(* Logix 5000 AddOnInstructionDefinition export YAI_Assy_170_22_23_EIP_Hz; software revision 21.03 *)

ADD_ON_INSTRUCTION YAI_Assy_170_22_23_EIP_Hz   (* revision 1.0, vendor Yaskawa America, Inc. *)
// YAI Assembly 170 and 22/23
// Help:
// This add-on instruction is for use with input assembly 170 and output assemblies 22/23.
// Node_Input_Assy is defined as the node's input assembly integer array.
// Node_Output_Assy is defined as the node's output assembly integer array.
// Torque limit/reference, torque compensation and torque output variables are only available with A1000.
VAR_IN_OUT
   Node_Input_Assy : AB:ETHERNET_MODULE_INT_24Bytes:I:0; {required}   // Input assembly words
   Node_Output_Assy : AB:ETHERNET_MODULE_INT_6Bytes:O:0; {required}   // Output assembly words
END_VAR
VAR_OUTPUT
   Running : BOOL; {access Read Only, visible}   // Drive running forward status bit
   ZSP : BOOL; {access Read Only, visible}   // Drive zero speed status bit
   RunningRev : BOOL; {access Read Only, visible}   // Drive running reverse status bit
   Reset : BOOL; {access Read Only, visible}   // Drive reset command status bit
   At_Speed : BOOL; {access Read Only, visible}   // Drive at commanded speed status bit
   Ready : BOOL; {access Read Only, visible}   // Drive ready status bit
   Alarm : BOOL; {access Read Only, visible}   // Drive alarm status bit
   Faulted : BOOL; {access Read Only, visible}   // Drive faulted status bit
   OPE : BOOL; {access Read Only}   // OPE alarm/fault present
   UV : BOOL; {access Read Only}   // Drive in UV (undervoltage) state status bit
   NetCtrlStatus : BOOL; {access Read Only, visible}   // Drive network run source status bit (1 = source coming from network)
   MFO_1_Status : BOOL; {access Read Only, visible}   // Drive multi-function output 1 (M1-M2 for A/P1000, MA/MB/MC for V1000) status
   MFO_2_Status : BOOL; {access Read Only, visible}   // Drive multi-function output 1 (M3-M4 for A/P1000, P1 for V1000) status
   MFO_3_Status : BOOL; {access Read Only, visible}   // Drive multi-function output 1 (M5-M6 for A/P1000, P2 for V1000) status
   ZSV : BOOL; {access Read Only, visible}   // Drive zero servo completed status bit
   Motor_Speed : REAL; {access Read Only, visible}   // Motor speed in Hz (xx.xx resolution)
   Custom_In_1 : INT; {access Read Only}
   Custom_In_2 : INT; {access Read Only}
   Custom_In_3 : INT; {access Read Only}
   Custom_In_4 : INT; {access Read Only}
   Custom_In_5 : INT; {access Read Only}
   Custom_In_6 : INT; {access Read Only}
   Custom_In_7 : INT; {access Read Only}
   Custom_In_8 : INT; {access Read Only}
   Custom_In_9 : INT; {access Read Only}
   Custom_In_10 : INT; {access Read Only}
END_VAR
VAR_INPUT
   Torq_Ref_Limit : REAL; {visible}   // Torque reference/limit (A1000 only) Engineering Units
   RunRev : BOOL; {visible}   // Reverse run command
   RunFwd : BOOL; {visible}   // Forward run command
   Net_Ref : BOOL;   // Network reference bit to switch between b1-01 setting and network.
   Net_Control : BOOL;   // Network control bit to switch between b1-02 setting and network.
   Motor_Rated_Torq : REAL := 100.0; {visible}   // Motor rated torque (Engineering units)
   Freq_Ref : REAL; {visible}   // Frequency reference command in Hz (xx.xx resolution)
   FaultReset : BOOL; {visible}   // Fault reset command
END_VAR
VAR
   FRef_Convert : DINT;
   FOut_Convert : REAL;
   FOut_Temp : REAL;
   TRef_Convert : INT;
   TComp_Convert : INT;
   TOut_Convert : REAL;
   TOut_Temp : REAL;
   IOut_Temp : REAL;
   IOut_Convert : REAL;
   AO1_Convert : INT;
   AO2_Convert : INT;
   Motor_Speed_Temp : REAL;
   Motor_Speed_Convert : REAL;
   Freq_Cmd_Temp : REAL;
   Freq_Cmd_Convert : REAL;
   AI1_Temp : REAL;
   AI1_Convert : REAL;
   AI2_Temp : REAL; {access None}
   AI2_Convert : REAL; {access None}
   AI3_Temp : REAL; {access None}
   AI3_Convert : REAL; {access None}
END_VAR

ROUTINE Logic   (* ladder *)
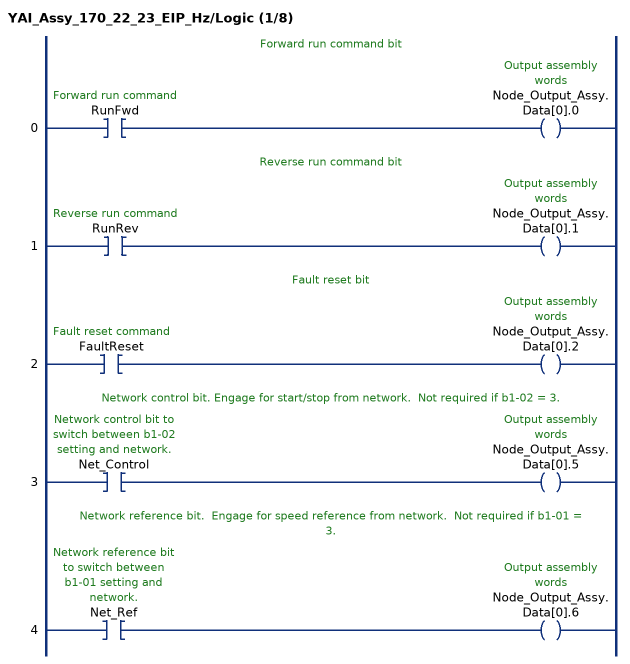
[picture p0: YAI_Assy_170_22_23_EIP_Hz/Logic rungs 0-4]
   // Forward run command bit
   0: XIC(RunFwd)OTE(Node_Output_Assy.Data[0].0);
   // Reverse run command bit
   1: XIC(RunRev)OTE(Node_Output_Assy.Data[0].1);
   // Fault reset bit
   2: XIC(FaultReset)OTE(Node_Output_Assy.Data[0].2);
   // Network control bit. Engage for start/stop from network.  Not required if b1-02 = 3.
   3: XIC(Net_Control)OTE(Node_Output_Assy.Data[0].5);
   // Network reference bit.  Engage for speed reference from network.  Not required if b1-01 = 3.
   4: XIC(Net_Ref)OTE(Node_Output_Assy.Data[0].6);
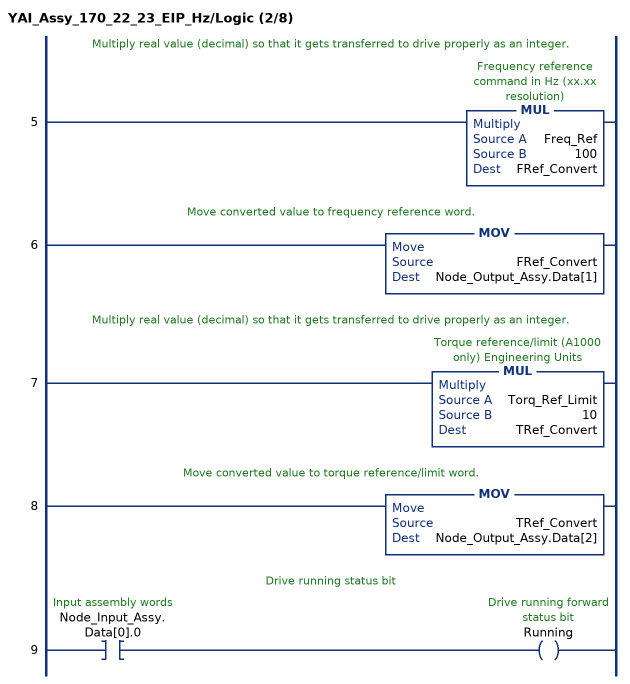
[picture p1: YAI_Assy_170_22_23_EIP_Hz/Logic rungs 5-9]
   // Multiply real value (decimal) so that it gets transferred to drive properly as an integer.
   5: MUL(Freq_Ref,100,FRef_Convert);
   // Move converted value to frequency reference word.
   6: MOV(FRef_Convert,Node_Output_Assy.Data[1]);
   // Multiply real value (decimal) so that it gets transferred to drive properly as an integer.
   7: MUL(Torq_Ref_Limit,10,TRef_Convert);
   // Move converted value to torque reference/limit word.
   8: MOV(TRef_Convert,Node_Output_Assy.Data[2]);
   // Drive running status bit
   9: XIC(Node_Input_Assy.Data[0].0)OTE(Running);
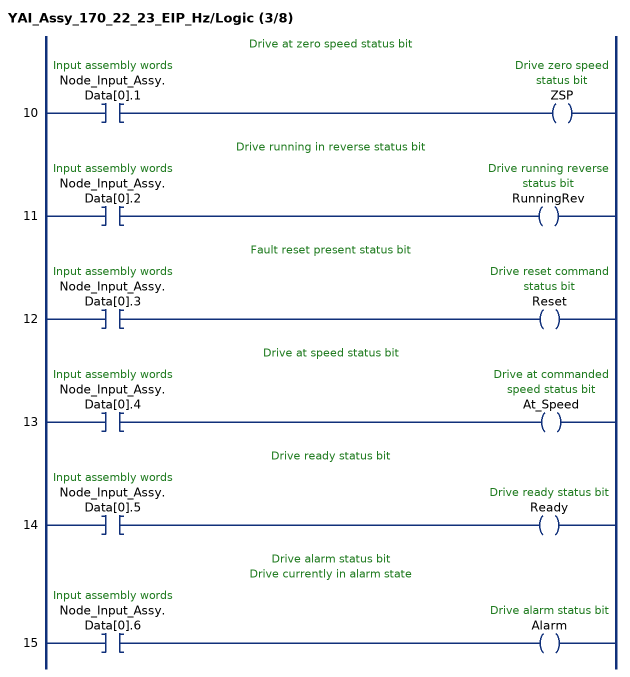
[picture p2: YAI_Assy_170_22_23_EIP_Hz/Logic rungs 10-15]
   // Drive at zero speed status bit
   10: XIC(Node_Input_Assy.Data[0].1)OTE(ZSP);
   // Drive running in reverse status bit
   11: XIC(Node_Input_Assy.Data[0].2)OTE(RunningRev);
   // Fault reset present status bit
   12: XIC(Node_Input_Assy.Data[0].3)OTE(Reset);
   // Drive at speed status bit
   13: XIC(Node_Input_Assy.Data[0].4)OTE(At_Speed);
   // Drive ready status bit
   14: XIC(Node_Input_Assy.Data[0].5)OTE(Ready);
   // Drive alarm status bit
   // Drive currently in alarm state
   15: XIC(Node_Input_Assy.Data[0].6)OTE(Alarm);
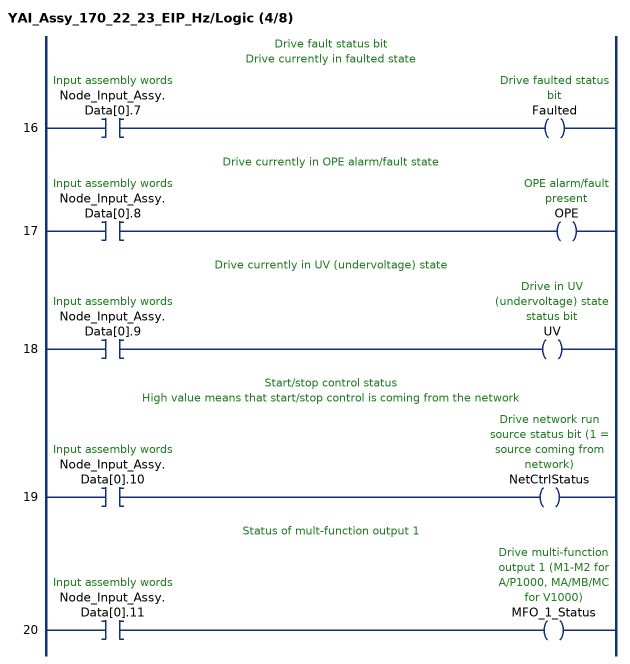
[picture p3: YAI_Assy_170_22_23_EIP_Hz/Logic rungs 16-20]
   // Drive fault status bit
   // Drive currently in faulted state
   16: XIC(Node_Input_Assy.Data[0].7)OTE(Faulted);
   // Drive currently in OPE alarm/fault state
   17: XIC(Node_Input_Assy.Data[0].8)OTE(OPE);
   // Drive currently in UV (undervoltage) state
   18: XIC(Node_Input_Assy.Data[0].9)OTE(UV);
   // Start/stop control status
   // High value means that start/stop control is coming from the network
   19: XIC(Node_Input_Assy.Data[0].10)OTE(NetCtrlStatus);
   // Status of mult-function output 1
   20: XIC(Node_Input_Assy.Data[0].11)OTE(MFO_1_Status);
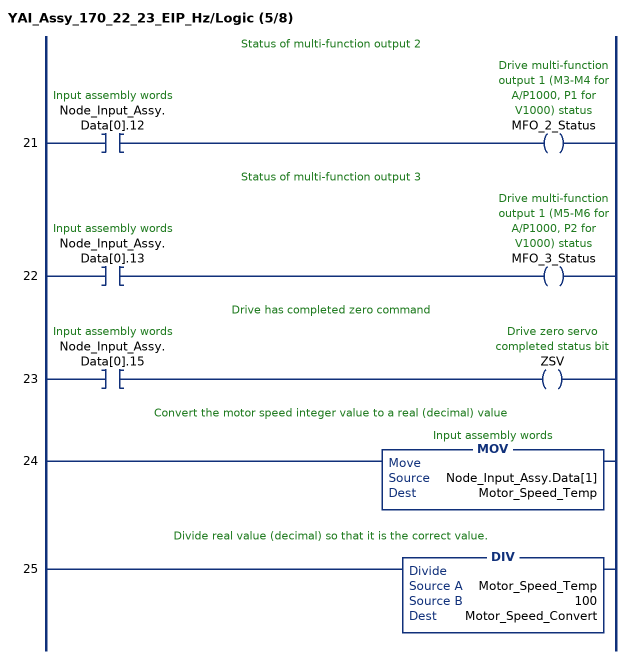
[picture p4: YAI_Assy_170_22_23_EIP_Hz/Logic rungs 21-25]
   // Status of multi-function output 2
   21: XIC(Node_Input_Assy.Data[0].12)OTE(MFO_2_Status);
   // Status of multi-function output 3
   22: XIC(Node_Input_Assy.Data[0].13)OTE(MFO_3_Status);
   // Drive has completed zero command
   23: XIC(Node_Input_Assy.Data[0].15)OTE(ZSV);
   // Convert the motor speed integer value to a real (decimal) value
   24: MOV(Node_Input_Assy.Data[1],Motor_Speed_Temp);
   // Divide real value (decimal) so that it is the correct value.
   25: DIV(Motor_Speed_Temp,100,Motor_Speed_Convert);
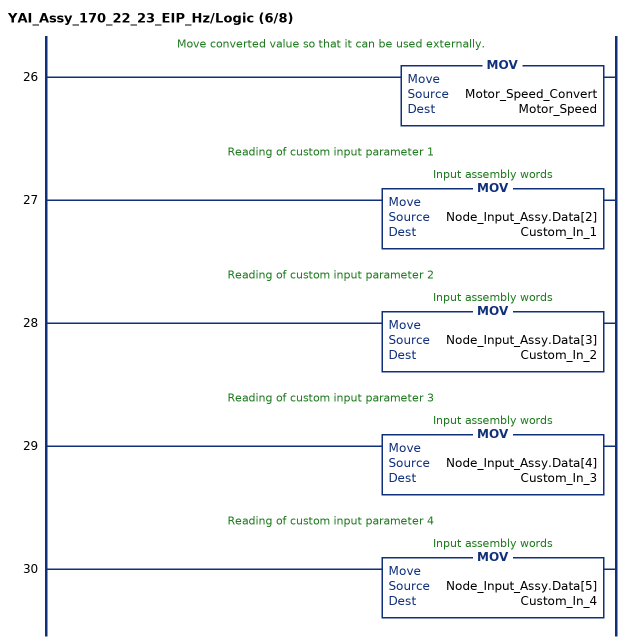
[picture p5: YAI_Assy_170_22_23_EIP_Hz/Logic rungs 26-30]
   // Move converted value so that it can be used externally.
   26: MOV(Motor_Speed_Convert,Motor_Speed);
   // Reading of custom input parameter 1
   27: MOV(Node_Input_Assy.Data[2],Custom_In_1);
   // Reading of custom input parameter 2
   28: MOV(Node_Input_Assy.Data[3],Custom_In_2);
   // Reading of custom input parameter 3
   29: MOV(Node_Input_Assy.Data[4],Custom_In_3);
   // Reading of custom input parameter 4
   30: MOV(Node_Input_Assy.Data[5],Custom_In_4);
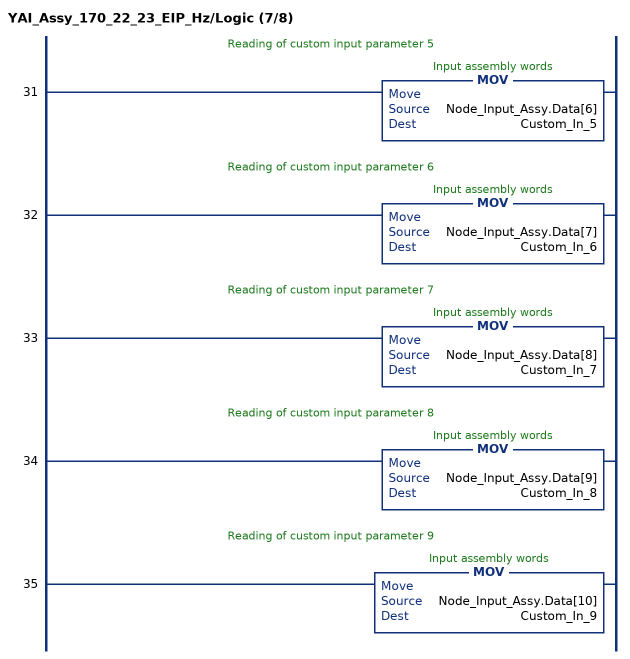
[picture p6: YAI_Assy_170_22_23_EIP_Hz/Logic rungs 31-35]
   // Reading of custom input parameter 5
   31: MOV(Node_Input_Assy.Data[6],Custom_In_5);
   // Reading of custom input parameter 6
   32: MOV(Node_Input_Assy.Data[7],Custom_In_6);
   // Reading of custom input parameter 7
   33: MOV(Node_Input_Assy.Data[8],Custom_In_7);
   // Reading of custom input parameter 8
   34: MOV(Node_Input_Assy.Data[9],Custom_In_8);
   // Reading of custom input parameter 9
   35: MOV(Node_Input_Assy.Data[10],Custom_In_9);
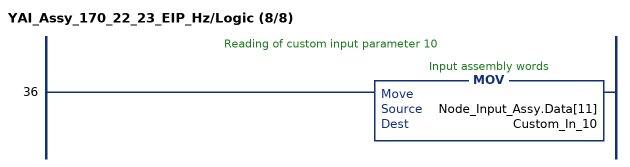
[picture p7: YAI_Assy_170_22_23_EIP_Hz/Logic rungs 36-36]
   // Reading of custom input parameter 10
   36: MOV(Node_Input_Assy.Data[11],Custom_In_10);
END_ROUTINE
END_ADD_ON_INSTRUCTION
